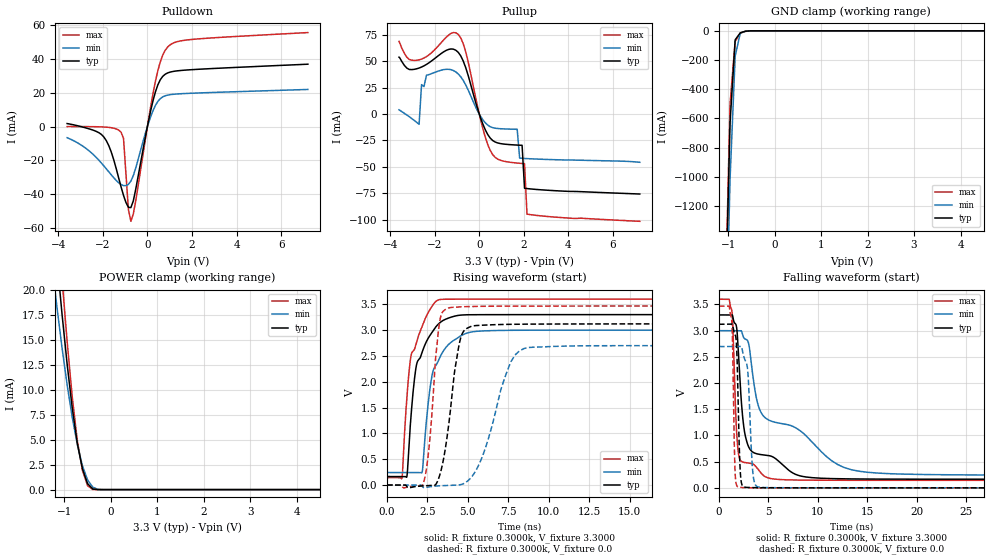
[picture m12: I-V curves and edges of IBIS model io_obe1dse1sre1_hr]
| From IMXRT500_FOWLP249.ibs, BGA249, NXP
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[Model] io_obe1dse1sre1_hr
|   Model io_obe1dse1sre1_hr
| Library cells for typ/min/max conditions are connected as defined below:
|  pad - External Pad
|  ipp_do - Core Input
|  ipp_obe - Output Buffer Enable
|  REFH3V3 - vdd1v8
|  REFL3V3 - vdd1v8
|  gnde - gnde
|  ipp_dse - vdd
|  ipp_ina235_3v - NC
|  ipp_ina40_3v - NC
|  ipp_ina_mux - NC
|  ipp_ind - NC
|  ipp_ind_1p8v - NC
|  ipp_ind_3v - NC
|  ipp_sre - vdd
|  vdd - vdd
|  vdd1v8 - vdd1v8
|  vdda - vdde3v3
|  vdde3v3 - vdde3v3
| All other pins connected to ground
Model_type I/O
Polarity   Non-Inverting
Enable   Active-High
Vinl =   0.9900V
Vinh =   2.3100V
Vmeas =  1.6500V
Cref =   25.0000pF
Rref =   0.5000k
Vref =   0.0V
C_comp   1.8291pF   1.7592pF   1.9119pF
[Temperature Range]   25.0000   0.1250k   -40.0000
[Voltage Range]   3.3000V   3.0000V   3.6000V
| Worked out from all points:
|   slope of the pulldown table from 0 to 0.495 V, typ, clamps not added: 19.4 ohm
|   slope of the pullup table from 0 to 0.495 V, typ, clamps not added: 21.6 ohm
|   GND clamp passes 1 mA (typ) near -0.55 V on its own axis
|   POWER clamp passes 1 mA (typ) near -0.53 V on its own axis
|   rising waveform, R_fixture 0.3000k, V_fixture 3.3000: 20-80 % time 926ps typ, 913ps min, 914ps max; typ from 0.165 V to 3.3 V
|   rising waveform, R_fixture 0.3000k, V_fixture 0.0: 20-80 % time 772ps typ, 1.5ns min, 521ps max; typ from 0 V to 3.12 V
|   falling waveform, R_fixture 0.3000k, V_fixture 3.3000: 20-80 % time 1.04ns typ, 6.59ns min, 434ps max; typ from 3.3 V to 0.165 V
|   falling waveform, R_fixture 0.3000k, V_fixture 0.0: 20-80 % time 255ps typ, 386ps min, 192ps max; typ from 3.12 V to 0 V
[Pulldown]
|Voltage   I(typ)   I(min)   I(max)
-3.6V     1.86mA     -6.52mA    90uA
-1.95V    -6.13mA    -23.22mA   -180uA
-1.62V    -14.97mA   -28.49mA   -600uA
-1.18V    -35.64mA   -34.24mA   -3.216mA
-1.07V    -40.67mA   -34.88mA   -6.929mA
-850mV    -47.74mA   -34.14mA   -49.09mA
-740mV    -47.9mA    -32.2mA    -56.02mA
-520mV    -36.89mA   -24.41mA   -43.8mA
360mV     20.57mA    12.57mA    26.82mA
580mV     27.83mA    16.63mA    38.42mA
910mV     31.85mA    18.72mA    47.2mA
7.2V      37.02mA    22.06mA    55.76mA
[Pullup]
|Voltage   I(typ)   I(min)   I(max)
-3.6V     54.05mA    4.09mA     68.98mA
-2.7V     43.72mA    -9.663mA   51.48mA
-2.59V    44.67mA    27.96mA    52.2mA
-2.37V    47.15mA    36.87mA    54.55mA
-940mV    58.52mA    38.04mA    75.65mA
490mV     -22.73mA   -11.94mA   -34.44mA
1.7V      -29.38mA   -14.4mA    -46.43mA
1.81V     -29.5mA    -41.73mA   -46.65mA
1.92V     -29.61mA   -41.91mA   -46.85mA
2.03V     -70.35mA   -42.07mA   -47.04mA
2.14V     -70.63mA   -42.21mA   -94.89mA
7.2V      -75.83mA   -45.7mA    -101.7mA
[GND_clamp]
|Voltage   I(typ)   I(min)   I(max)
-3.6V     -46.64A    -46.27A    -48.09A
-1.07V    -2.038A    -2.424A    -1.965A
-960mV    -629.9mA   -1.012A    -499.2mA
-850mV    -61.62mA   -174.1mA   -72.03mA
-740mV    -13.6mA    -15.66mA   -16.3mA
-630mV    -2.66mA    -3.244mA   -3.912mA
-410mV    -9.358uA   -49.22uA   -3.515uA
7.2V      0A         0A         0A
[POWER_clamp]
|Voltage   I(typ)   I(min)   I(max)
-3.6V     129.4mA    109.3mA    143.3mA
-1.27V    28.99mA    22.71mA    35.27mA
-1.16V    23.09mA    18.31mA    28mA
-1.05V    17.57mA    14.21mA    21.12mA
-940mV    12.56mA    10.49mA    14.82mA
-830mV    8.174mA    7.224mA    9.263mA
-720mV    4.592mA    4.483mA    4.857mA
-610mV    2.058mA    2.37mA     1.909mA
-500mV    597.2uA    970.5uA    391.6uA
-390mV    63.24uA    245.6uA    14.23uA
-170mV    54.62nA    1.775uA    12.62nA
7.2V      0A         0A         0A
[Ramp]
| variable   typ   min   max
dV/dt_r  0.8854/1.0712n   0.6599/2.0811n   1.3657/0.8309n
dV/dt_f  1.0033/7.7968n   0.5950/11.3153n   1.4811/4.7592n
R_load = 50.0000
[Rising Waveform]
R_fixture= 0.3000k
V_fixture= 3.3000
V_fixture_min= 3.0000
V_fixture_max= 3.6000
|time   V(typ)   V(min)   V(max)
0s        164.8mV    242.6mV    143.9mV
922.3ps   164.8mV    242.6mV    132.4mV
1.225ns   159.2mV    242.6mV    1.675V
1.469ns   1.27V      242.6mV    2.476V
1.713ns   2.091V     242.6mV    2.64V
2.163ns   2.563V     241.5mV    3.061V
2.761ns   2.944V     2.079V     3.451V
3.503ns   3.193V     2.604V     3.597V
9.297ns   3.3V       2.999V     3.6V
500ns     3.3V       3V         3.6V
[Rising Waveform]
R_fixture= 0.3000k
V_fixture= 0.0
V_fixture_min= 0.0
V_fixture_max= 0.0
|time   V(typ)   V(min)   V(max)
0s        114.1nV    649.7nV    480nV
2.219ns   -16.28mV   -42mV      9.163mV
2.61ns    -9.915mV   -34.79mV   755.2mV
3.077ns   41.81mV    -18.35mV   2.66V
3.421ns   386.7mV    -11.99mV   3.343V
4.499ns   2.777V     3.984mV    3.449V
5.321ns   3.082V     194.3mV    3.459V
7.914ns   3.114V     2.517V     3.465V
11.31ns   3.119V     2.693V     3.466V
500ns     3.122V     2.696V     3.467V
[Falling Waveform]
R_fixture= 0.3000k
V_fixture= 3.3000
V_fixture_min= 3.0000
V_fixture_max= 3.6000
|time   V(typ)   V(min)   V(max)
0s        3.3V       3V         3.6V
1.315ns   3.301V     3V         3.37V
1.771ns   3.081V     3V         1.123V
2.101ns   2.158V     2.999V     553.9mV
3.021ns   776.9mV    2.74V      473.4mV
4.17ns    636.8mV    1.473V     302.6mV
6.605ns   410.8mV    1.219V     154.9mV
12.67ns   172.2mV    387.8mV    144.4mV
22.53ns   165.1mV    250.5mV    143.9mV
500ns     164.8mV    242.6mV    143.9mV
[Falling Waveform]
R_fixture= 0.3000k
V_fixture= 0.0
V_fixture_min= 0.0
V_fixture_max= 0.0
|time   V(typ)   V(min)   V(max)
0s        3.122V     2.696V     3.467V
1.289ns   3.123V     2.696V     3.211V
1.589ns   2.937V     2.696V     562.5mV
1.715ns   2.872V     2.696V     106.7mV
2.153ns   326.6mV    2.699V     9.343mV
2.563ns   15.29mV    2.475V     4.215mV
2.943ns   7.186mV    2.168V     2.411mV
3.509ns   3.896mV    173.3mV    1.287mV
4.701ns   1.553mV    6.315mV    536.8uV
500ns     529.9nV    1.199uV    1.107uV
